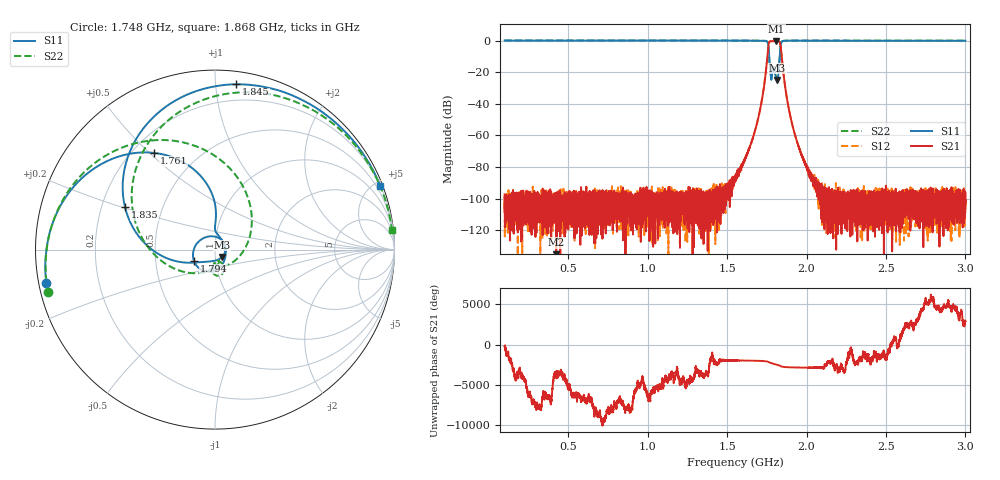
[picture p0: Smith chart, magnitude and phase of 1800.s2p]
# Hz S DB R 50
! Planar, S50180, 20087770, 20.1.2/1
! Date: 23.06.2021 14:47:52
! Data: Format (Calibration Info)
! Freq	S11:dB/Ang(F2)	S21:dB/Ang(F2)	S12:dB/Ang(F2)	S22:dB/Ang(F2)
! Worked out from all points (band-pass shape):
!   8991 points, 100 MHz to 3 GHz, reference 50 ohm
!   highest |S21| = -0.35 dB at 1.811 GHz (marker M1); lowest = -140.3 dB at 424.8 MHz (marker M2)
!   |S21| within 3 dB of the highest: 1.76 GHz to 1.837 GHz (76.25 MHz wide, 4.24 % of centre)
!   lowest |S11| = -25.0 dB at 1.816 GHz (marker M3), VSWR 1.12, Z = 53.9 - j4.4 ohm
!   |S11| at or under -10 dB: 1.765 GHz to 1.831 GHz (66.07 MHz wide, 3.67 % of centre)
!   |S22| runs from -24.0 to 0.0 dB; largest |S21 - S12| = 0.0029
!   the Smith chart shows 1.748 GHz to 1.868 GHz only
!   S11 on the Smith chart (normalised r, x): 1.748 GHz: 0.02, -0.10; 1.761 GHz: 0.29, +0.52; 1.794 GHz: 0.78, -0.10; 1.835 GHz: 0.30, +0.21; 1.845 GHz: 0.08, +1.13; 1.868 GHz: 0.20, +5.37
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1e8  0.02 153.9  -97.15 -153.0  -106.35 -9.0  0.01 150.1
2.558065e8  -0.02 116.3  -106.55 29.5  -105.98 -83.7  -0.01 108.9
4.248387e8  -0.01 81.6  -140.32 -47.8  -99.44 -79.9  -0.00 72.6
5.835484e8  -0.01 55.2  -103.42 -134.9  -119.80 -76.2  0.01 45.9
1.066774e9  -0.00 -5.1  -100.58 -33.6  -100.90 80.4  0.04 -11.1
1.55e9  -0.02 -60.4  -86.92 -146.9  -86.52 -146.0  0.02 -61.4
1.597742e9  -0.02 -69.1  -78.16 -154.1  -78.73 -154.2  -0.01 -69.1
1.663226e9  -0.05 -86.7  -61.17 -177.2  -61.24 -177.1  0.03 -84.5
1.722258e9  -0.11 -122.6  -35.84 148.2  -35.84 148.1  -0.09 -117.5
1.747742e9  -0.37 -168.7  -16.34 100.1  -16.35 100.1  -0.35 -165.7
1.760645e9  -3.93 122.1  -3.22 20.7  -3.23 20.6  -4.07 107.0
1.777742e9  -24.63 32.9  -0.39 -116.8  -0.40 -116.8  -23.55 -87.4
1.794194e9  -17.55 -152.6  -0.41 149.0  -0.43 148.9  -16.75 -86.4
1.810968e9  -24.37 17.5  -0.35 57.0  -0.36 56.9  -23.54 -83.8
1.815806e9  -24.95 -46.1  -0.36 28.9  -0.38 28.8  -24.01 -72.9
1.835161e9  -5.12 154.7  -2.40 -115.0  -2.40 -115.2  -5.23 148.0
1.845484e9  -0.65 82.7  -11.60 167.4  -11.61 167.3  -0.65 66.3
1.868065e9  -0.12 21.1  -30.94 105.5  -30.95 105.4  -0.07 6.3
1.951613e9  -0.02 -34.2  -67.37 53.4  -67.28 51.3  -0.00 -42.0
2.033548e9  -0.04 -52.8  -88.15 40.1  -84.77 43.2  -0.01 -58.0
2.516774e9  -0.08 -101.8  -102.58 51.2  -97.84 -14.6  -0.05 -101.7
3e9  -0.12 -138.0  -101.55 40.3  -97.42 -54.4  -0.08 -135.3
